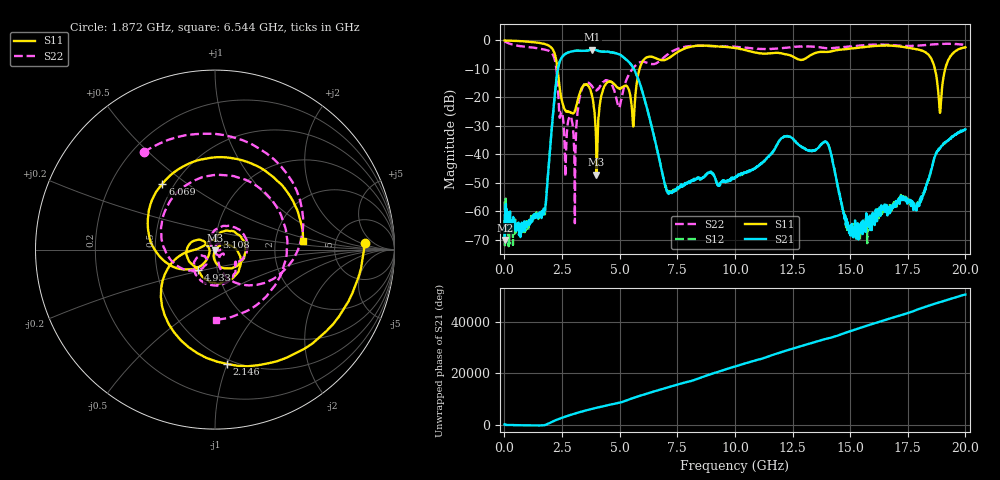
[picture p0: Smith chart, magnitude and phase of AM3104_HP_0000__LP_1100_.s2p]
!Created with skrf (http://scikit-rf.org).
# Hz S RI R 50.0
!freq ReS11 ImS11 ReS21 ImS21 ReS12 ImS12 ReS22 ImS22
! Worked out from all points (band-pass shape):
!   1601 points, 10 MHz to 20 GHz, reference 50 ohm
!   highest |S21| = -3.16 dB at 3.808 GHz (marker M1); lowest = -70.0 dB at 22.49 MHz (marker M2)
!   |S21| within 3 dB of the highest: 2.473 GHz to 5.205 GHz (2.732 GHz wide, 71.2 % of centre)
!   lowest |S11| = -47.2 dB at 3.996 GHz (marker M3), VSWR 1.01, Z = 50 - j0.437 ohm
!   |S11| at or under -10 dB: 2.306 GHz to 5.864 GHz (3.559 GHz wide, 87.1 % of centre); 18.68 GHz to 19.12 GHz (442.7 MHz wide, 2.34 % of centre)
!   |S22| runs from -64.1 to -0.2 dB; largest |S21 - S12| = 0.0057
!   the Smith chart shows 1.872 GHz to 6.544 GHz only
!   S11 on the Smith chart (normalised r, x): 1.872 GHz: 10, +3; 2.146 GHz: 0.46, -1.00; 3.108 GHz: 1.01, +0.14; 4.933 GHz: 0.81, -0.19; 6.069 GHz: 0.43, +0.41; 6.544 GHz: 2.89, +0.36
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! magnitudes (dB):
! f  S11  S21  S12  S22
! 10 MHz  0.0  -63.5  -56.6  -0.2
! 22.49 MHz  0.0  -70.0  -72.0  -0.3
! 1.872 GHz  -1.6  -49.2  -48.8  -3.4
! 2.146 GHz  -3.9  -22.6  -22.6  -5.7
! 2.609 GHz  -24.1  -4.9  -4.9  -35.9
! 3.108 GHz  -23.2  -3.6  -3.6  -32.7
! 3.346 GHz  -16.8  -3.6  -3.7  -17.5
! 3.808 GHz  -19.5  -3.2  -3.1  -16.1
! 3.996 GHz  -47.2  -3.4  -3.4  -17.4
! 4.933 GHz  -16.7  -4.7  -4.7  -22.8
! 5.582 GHz  -29.8  -9.5  -9.5  -9.8
! 6.069 GHz  -6.6  -20.3  -20.3  -7.5
! 6.544 GHz  -6.1  -35.5  -35.5  -8.1
! 6.682 GHz  -6.6  -40.3  -40.3  -7.6
! 7.169 GHz  -6.0  -53.4  -53.0  -4.4
! 10.01 GHz  -2.6  -48.3  -48.0  -2.2
! 13.34 GHz  -4.9  -38.7  -38.8  -2.2
! 14.04 GHz  -4.0  -36.5  -36.4  -2.8
! 14.98 GHz  -2.9  -66.8  -65.2  -2.1
! 16.68 GHz  -1.8  -58.9  -59.5  -1.5
! 18.9 GHz  -25.4  -37.8  -37.8  -1.2
! 20 GHz  -2.4  -31.2  -31.3  -1.5
